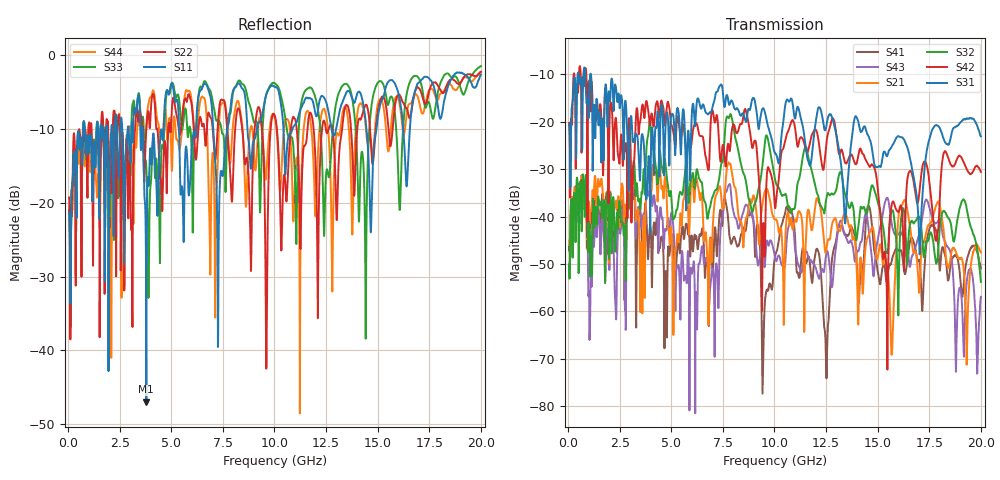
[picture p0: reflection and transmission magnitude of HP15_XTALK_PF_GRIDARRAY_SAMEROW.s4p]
# MHz S MA R 50.00
! FREQ  S11  S12  S13  S14
!  S21  S22  S23  S24
!  S31  S32  S33  S34
!  S41  S42  S43  S44
!  MAG  ANG  MAG  ANG  MAG  ANG  MAG  ANG
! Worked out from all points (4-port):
!   1996 points, 50 MHz to 20 GHz, reference 50 ohm
!   strongest paths, dB at 50 MHz, 5.04 GHz, 10.03 GHz, 15.02 GHz, 20 GHz:
!     S31: -20.7, -18.3, -26.7, -29.5, -23.1
!     S42: -20.2, -21.0, -38.2, -34.8, -30.6
!     S32: -50.1, -38.6, -32.3, -37.2, -53.8
!     S21: -45.9, -45.8, -40.6, -48.2, -47.6
!     S43: -50.3, -39.5, -48.8, -44.5, -56.9
!     S41: -47.1, -43.8, -48.4, -52.0, -50.9
!   lowest |S11| = -46.9 dB at 3.79 GHz (marker M1), VSWR 1.01, Z = 49.6 - j0.266 ohm
!   |S11| at or under -10 dB: start of sweep to 720.8 MHz; 3.609 GHz to 4.63 GHz (1.021 GHz wide, 24.8 % of centre); 5.378 GHz to 6.201 GHz (823.3 MHz wide, 14.2 % of centre)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
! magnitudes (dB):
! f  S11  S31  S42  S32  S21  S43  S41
! 50 MHz  -21.4  -20.7  -20.2  -50.1  -45.9  -50.3  -47.1
! 3.79 GHz  -46.9  -36.4  -15.6  -26.2  -34.3  -36.2  -39.6
! 8.6 GHz  -6.2  -19.9  -17.4  -32.2  -40.8  -37.6  -43.1
! 9.46 GHz  -7.3  -17.1  -41.5  -27.6  -36.2  -47.1  -68.8
! 12.84 GHz  -10.9  -19.7  -19.3  -35.4  -40.9  -52.9  -47.5
! 15.43 GHz  -4.1  -27.2  -53.1  -47.7  -50.1  -36.1  -53.9
! 20 GHz  -2.7  -23.1  -30.6  -53.8  -47.6  -56.9  -50.9
